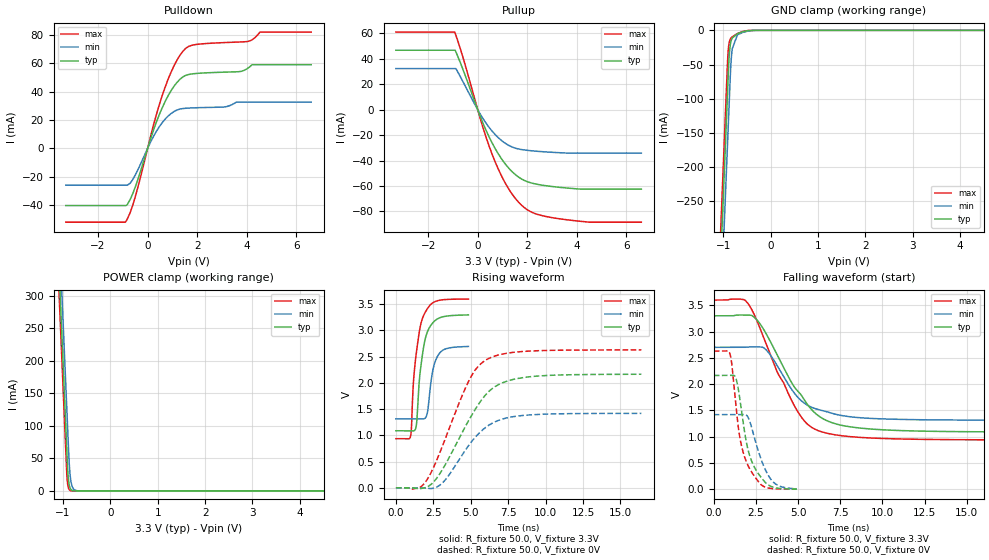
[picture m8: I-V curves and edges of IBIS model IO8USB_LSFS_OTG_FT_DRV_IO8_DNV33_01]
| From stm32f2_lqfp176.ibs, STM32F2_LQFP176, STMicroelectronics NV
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| *** New cell (Generated with 5.14beta1 (Sep 20 2010 13:23:23))
[Model]   IO8USB_LSFS_OTG_FT_DRV_IO8_DNV33_01
Model_type 3-state
Polarity   Non-Inverting
Enable   Active-Low
| CAP_THRESHOLD on pad DPV33 is "CMOS" :
| Rising=10.0% of vddio   Falling=90.0% of vddio
| C_comp min and max val. don't necessarily correlate with the min and max pvt
| but are the smallest and greatest pad capacitance found.
| var   typ   min   max
C_comp   5.85475pF  5.58530pF  6.39105pF
Vmeas = 1.65V   | Reference voltage for timing measurements
Cref  = 400.0pF   | Timing specification test load capacitance value
Rref  = 1.0MOhm   | Timing specification test load resistance value
Vref  = 1.65V   | Timing specification test load voltage
[Model Spec]
| variable   typ   min   max
[Temperature Range] 25.0 125.0 -40.0
| variable   typ   min   max
[Voltage Range] 3.3V 2.7V 3.6V
| variable   typ   min   max
[POWER Clamp Reference] 3.3V 2.7V 3.6V
| variable   typ   min   max
[GND Clamp Reference] 0V 0V 0V
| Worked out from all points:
|   slope of the pulldown table from 0 to 0.495 V, typ, clamps not added: 20 ohm
|   slope of the pullup table from 0 to 0.495 V, typ, clamps not added: 21.7 ohm
|   GND clamp passes 1 mA (typ) near -0.51 V on its own axis
|   POWER clamp passes 1 mA (typ) near -0.81 V on its own axis
|   rising waveform, R_fixture 50.0, V_fixture 3.3V: 20-80 % time 522ps typ, 457ps min, 538ps max; typ from 1.09 V to 3.3 V
|   falling waveform, R_fixture 50.0, V_fixture 3.3V: 20-80 % time 2.48ns typ, 1.97ns min, 2.26ns max; typ from 3.3 V to 1.09 V
|   rising waveform, R_fixture 50.0, V_fixture 0V: 20-80 % time 2.59ns typ, 2.28ns min, 2.26ns max; typ from 0 V to 2.17 V
|   falling waveform, R_fixture 50.0, V_fixture 0V: 20-80 % time 847ps typ, 908ps min, 768ps max; typ from 2.17 V to 0.002 V
[POWER Clamp]
-3.3V     4.11A      4.173A     4.072A
-1.09V    352.5mA    415.9mA    314.5mA
-1.05V    284.5mA    347.9mA    246.5mA
-1.01V    216.5mA    279.9mA    178.5mA
-920mV    63.51mA    126.9mA    25.85mA
-900mV    31.51mA    92.9mA     9.552mA
-890mV    21.35mA    75.9mA     5.807mA
-870mV    9.804mA    44.01mA    2.146mA
-840mV    3.05mA     18.36mA    482.1uA
-780mV    295.2uA    3.193mA    24.34uA
-660mV    2.775uA    96uA       63.85nA
6.6V      0A         0A         0A
[GND Clamp]
-3.3V     -4.155A    -4.23A     -4.11A
-1.06V    -347.4mA   -421.9mA   -301.9mA
-940mV    -143.4mA   -217.9mA   -97.86mA
-910mV    -92.43mA   -166.9mA   -46.86mA
-890mV    -58.43mA   -132.9mA   -25.36mA
-880mV    -43.4mA    -115.9mA   -20.1mA
-860mV    -25.79mA   -81.93mA   -14.41mA
-840mV    -17.12mA   -51.2mA    -11.69mA
-820mV    -12.64mA   -32.88mA   -10.09mA
-700mV    -5.102mA   -6.6mA     -4.73mA
-230mV    -826nA     -13.68uA   -47.8nA
6.6V      45.45nA    5.674uA    302.2pA
| variable   typ   min   max
[Pullup Reference] 3.3V 2.7V 3.6V
| variable   typ   min   max
[Pulldown Reference] 0V 0V 0V
[Pullup]
-3.3V     46.81mA    32.38mA    61.09mA
-930mV    46.81mA    32.38mA    61.09mA
-880mV    45.47mA    32.38mA    58.55mA
-590mV    31.39mA    21.85mA    40.84mA
240mV     -11.89mA   -7.822mA   -15.87mA
590mV     -26.5mA    -17.07mA   -35.52mA
1.18V     -44.36mA   -27.27mA   -60.11mA
1.54V     -51.43mA   -30.39mA   -70.35mA
1.89V     -55.75mA   -31.69mA   -77.18mA
2.48V     -58.98mA   -32.83mA   -82.75mA
3.6V      -61.62mA   -34.07mA   -86.61mA
6.6V      -62.54mA   -34.07mA   -88.51mA
[Pulldown]
-3.3V     -40.26mA   -25.94mA   -51.99mA
-870mV    -40.25mA   -25.94mA   -51.33mA
-700mV    -35.92mA   -24.51mA   -45.06mA
-470mV    -25.89mA   -17.87mA   -32.39mA
240mV     12.97mA    8.52mA     16.62mA
590mV     28.62mA    18.11mA    37.2mA
1.07V     43.85mA    26mA       58.31mA
1.54V     51.42mA    28.24mA    70.48mA
2.01V     52.82mA    28.63mA    73.27mA
4.01V     56.01mA    32.56mA    75.18mA
4.53V     58.89mA    32.56mA    81.88mA
6.6V      58.89mA    32.56mA    81.88mA
[Ramp]
dV/dt_r 1.29886V/2.59061ns 851.30628mV/2.27686ns 1.57727V/2.25922ns
dV/dt_f 1.32782V/2.48146ns 831.60177mV/1.97086ns 1.59819V/2.25674ns
R_load = 50.0
| Removed startup time: 0s 0s 0s  .
| Removed end time: 4.842ns.
[Rising Waveform]
R_fixture   = 50.0
V_fixture   = 3.3V
V_fixture_min = 2.7V
V_fixture_max = 3.6V
0s        1.087V     1.314V     936.3mV
981ps     1.087V     1.314V     986.5mV
1.158ns   1.084V     1.314V     1.964V
1.305ns   1.119V     1.314V     2.437V
1.599ns   2.155V     1.313V     3.036V
1.912ns   2.779V     1.319V     3.322V
2.117ns   2.983V     1.455V     3.422V
2.47ns    3.147V     2.246V     3.527V
2.822ns   3.227V     2.529V     3.569V
4.844ns   3.296V     2.694V     3.598V
| Removed startup time: 0s 0s 0s  .
| Removed end time: 20.595ns.
[Falling Waveform]
R_fixture   = 50.0
V_fixture   = 3.3V
V_fixture_min = 2.7V
V_fixture_max = 3.6V
0s        3.3V       2.7V       3.6V
2.015ns   3.315V     2.707V     3.54V
2.485ns   3.246V     2.711V     3.262V
3.095ns   2.966V     2.655V     2.772V
4.82ns    1.927V     1.812V     1.564V
5.47ns    1.649V     1.616V     1.265V
6.205ns   1.398V     1.516V     1.113V
7.4ns     1.23V      1.414V     1.025V
9.455ns   1.142V     1.345V     972.5mV
20.61ns   1.087V     1.314V     936.7mV
| Removed startup time: 0s 0s 0s  .
| Removed end time: 16.385ns.
[Rising Waveform]
R_fixture   = 50.0
V_fixture   = 0V
V_fixture_min = 0V
V_fixture_max = 0V
0s        17.01nV    1.21uV     10.9nV
1.425ns   -14.35mV   46.03uV    -8.324mV
2.025ns   8.1mV      -6.303mV   129.7mV
3.165ns   375mV      109.1mV    835.6mV
4.905ns   1.306V     824.5mV    2.059V
5.46ns    1.568V     1.014V     2.303V
6.14ns    1.817V     1.181V     2.457V
7.28ns    2.02V      1.324V     2.559V
8.735ns   2.11V      1.385V     2.603V
16.4ns    2.165V     1.419V     2.629V
| Removed startup time: 0s 0s 0s  .
| Removed end time: 4.928ns.
[Falling Waveform]
R_fixture   = 50.0
V_fixture   = 0V
V_fixture_min = 0V
V_fixture_max = 0V
0s        2.165V     1.419V     2.629V
952ps     2.165V     1.419V     2.583V
1.074ns   2.168V     1.419V     2.367V
1.295ns   2.125V     1.418V     1.65V
1.556ns   1.69V      1.42V      965mV
1.915ns   924.8mV    1.415V     535.8mV
2.2ns     571.8mV    1.224V     348mV
2.826ns   217mV      551.6mV    81.63mV
3.354ns   59.26mV    202mV      15.98mV
4.93ns    1.806mV    7.46mV     964.9uV
